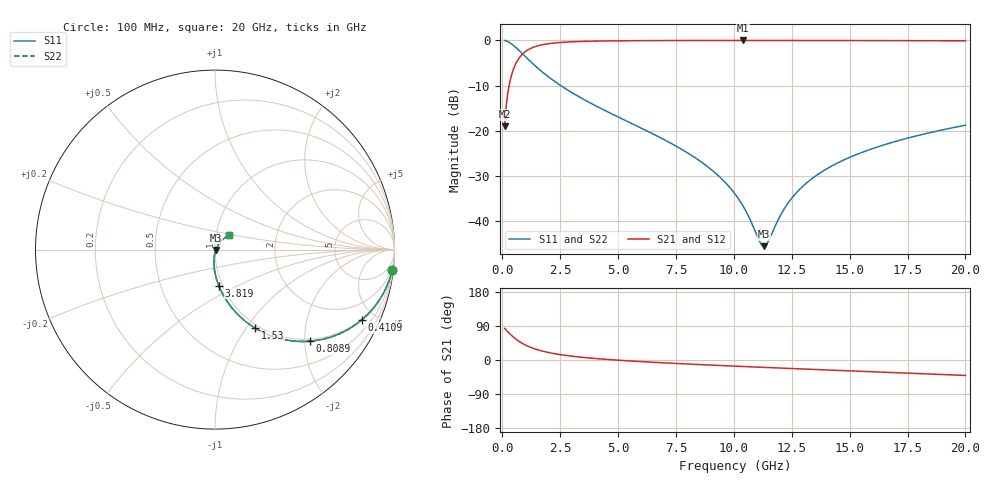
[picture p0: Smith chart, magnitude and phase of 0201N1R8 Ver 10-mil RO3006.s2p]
# GHz S MA R 50
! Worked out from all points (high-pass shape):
!   1601 points, 100 MHz to 20 GHz, reference 50 ohm
!   highest |S21| = -0.05 dB at 10.4 GHz (marker M1); lowest = -19.0 dB at 100 MHz (marker M2)
!   |S21| within 3 dB of the highest: 873.8 MHz to end of sweep
!   lowest |S11| = -45.5 dB at 11.29 GHz (marker M3), VSWR 1.01, Z = 50.5 - j0.193 ohm
!   |S11| at or under -10 dB: 2.522 GHz to end of sweep
!   |S22| runs from -45.5 to -0.1 dB; largest |S21 - S12| = 0
!   S11 on the Smith chart (normalised r, x): 100 MHz: 1, -17; 410.9 MHz: 0.95, -4.18; 808.9 MHz: 0.95, -2.12; 1.53 GHz: 0.95, -1.11; 3.819 GHz: 0.96, -0.40; 20 GHz: 1.16, +0.19
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0.1  0.9936 -6.6  0.1124 83.4  0.1124 83.4  0.9936 -6.6
0.274125  0.9549 -17.7  0.2963 72.2  0.2963 72.2  0.9549 -17.7
0.4109375  0.9062 -25.7  0.4218 64.3  0.4218 64.3  0.9062 -25.7
0.5850625  0.8326 -34.6  0.5525 55.3  0.5525 55.3  0.8326 -34.6
0.8089375  0.7352 -43.9  0.676 45.9  0.676 45.9  0.7352 -43.9
1.14475  0.6065 -54.5  0.7929 35.3  0.7929 35.3  0.6065 -54.5
1.530312  0.4927 -62.9  0.8676 26.9  0.8676 26.9  0.4927 -62.9
2.289  0.3473 -73.2  0.9347 16.3  0.9347 16.3  0.3473 -73.2
3.420812  0.2294 -81.8  0.9698 7.3  0.9698 7.3  0.2294 -81.8
3.818812  0.2019 -84.0  0.9757 5.0  0.9757 5.0  0.2019 -84.0
6.741625  0.08627 -93.8  0.9917 -6.8  0.9917 -6.8  0.08627 -93.8
8.7565  0.04231 -96.2  0.9941 -12.8  0.9941 -12.8  0.04231 -96.2
10.05  0.02012 -91.6  0.9945 -16.3  0.9945 -16.3  0.02012 -91.6
10.39825  0.01479 -86.8  0.9945 -17.2  0.9945 -17.2  0.01479 -86.8
11.10719  0.006055 -47.9  0.9944 -19.0  0.9944 -19.0  0.006055 -47.9
11.29375  0.005338 -21.0  0.9944 -19.5  0.9944 -19.5  0.005338 -21.0
11.46787  0.005895 4.4  0.9943 -20.0  0.9943 -20.0  0.005895 4.4
12.36337  0.01624 47.9  0.994 -22.2  0.994 -22.2  0.01624 47.9
13.37081  0.02966 54.2  0.9935 -24.7  0.9935 -24.7  0.02966 54.2
14.77625  0.04807 54.7  0.9925 -28.1  0.9925 -28.1  0.04807 54.7
16.69162  0.07269 52.2  0.9906 -32.8  0.9906 -32.8  0.07269 52.2
20  0.1155 45.9  0.9859 -40.7  0.9859 -40.7  0.1155 45.9
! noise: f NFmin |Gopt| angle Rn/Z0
0.1  0.0009657  0.9568  0.6896  0.005031
2.301  0.005358  0.826  4.396  0.006464
4.515  0.008286  0.7844  8.137  0.007855
6.729  0.01081  0.7578  11.88  0.008936
8.943  0.01311  0.7384  15.6  0.009852
11.14  0.01527  0.7234  19.27  0.01066
13.36  0.01735  0.7115  22.92  0.0114
15.57  0.01937  0.7019  26.53  0.01208
17.79  0.02135  0.6942  30.1  0.01273
20  0.0233  0.688  33.62  0.01334
